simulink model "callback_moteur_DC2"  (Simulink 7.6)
settings: Solver=ode15s  StartTime=0.0  StopTime=N  RelTol=1e-3
InitFcn:
  | % Durée de simulation et temps de l'échelon
  | N=2;
  | t0=N/2;
  | t1=3*N/4;
StopFcn:
  | close all
  | load vit_pos_mot_DC.mat
  | plotyy(x(1,:),x(2,:), x(1,:),x(3,:))
  | grid
  | title('Position et Vitesse d''un moteur DC')
  | gtext('Position (rad)')
  | gtext('Vitesse (rad/s)')
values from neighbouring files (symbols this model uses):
  K = 0.0005    [parametres.m]
  R = 4    [parametres.m]    (also in Prog_callbacks.m = 1000; oscillateur_dephasage.m = 1000; Calcul_Ampl_phase_A.m = 1; circuit_RLC_parallele_.m)
libraries: fl_lib x10, nesl_utility x4

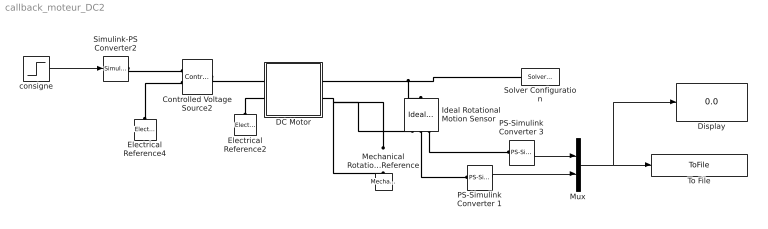
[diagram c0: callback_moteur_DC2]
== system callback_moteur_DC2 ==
  Controlled Voltage Source2 : fl_lib/Electrical/Electrical Sources/Controlled Voltage Source  DialogController=NetworkEngine.DynNeDlgSource  SystemSampleTime=-1  i_Log=off  v_Log=off  LocalVarNames=|current|voltage|power  LocalVarDescs=|Current (A)|Voltage (V)|Power (W)  LocalVarLogging=[0 0 0]
  DC Motor : Subsystem  LoadFcn=|
      | R=4; % Résistance d'induit             
      | L=1e-5; % Inductance d'induit          
      | K=0.0005; % paramètre électromagnétique
  Display : Display
  Electrical Reference2 : fl_lib/Electrical/Electrical Elements/Electrical Reference  DialogController=NetworkEngine.DynNeDlgSource  SystemSampleTime=-1  i_Log=off  LocalVarNames=|i  LocalVarDescs=|i  LocalVarLogging=[]
  Electrical Reference4 : fl_lib/Electrical/Electrical Elements/Electrical Reference  DialogController=NetworkEngine.DynNeDlgSource  SystemSampleTime=-1  i_Log=off  LocalVarNames=|i  LocalVarDescs=|i  LocalVarLogging=[]
  Ideal Rotational Motion Sensor : fl_lib/Mechanical/Mechanical Sensors/Ideal Rotational Motion Sensor  DialogController=NetworkEngine.DynNeDlgSource  SystemSampleTime=-1  offset=0 rad  w_Log=off  t_Log=off  phi_Log=off  LocalVarNames=|w|t|phi  LocalVarDescs=|w|t|phi  LocalVarLogging=[]
  Mechanical Rotational Reference : fl_lib/Mechanical/Rotational Elements/Mechanical Rotational Reference  DialogController=NetworkEngine.DynNeDlgSource  SystemSampleTime=-1  t_Log=off  LocalVarNames=|t  LocalVarDescs=|t  LocalVarLogging=[]
  Mux : Mux  Inputs=2
  PS-Simulink Converter 1 : nesl_utility/PS-Simulink Converter  DialogController=NetworkEngine.DynNeUtilDlgSource  SystemSampleTime=-1  PhysicalDomain=network_engine_domain  LeftPortType=input  RightPortType=output  SubClassName=ps_output  Unit=rpm  AffineConversion=off
  PS-Simulink Converter 3 : nesl_utility/PS-Simulink Converter  DialogController=NetworkEngine.DynNeUtilDlgSource  SystemSampleTime=-1  PhysicalDomain=network_engine_domain  LeftPortType=input  RightPortType=output  SubClassName=ps_output  Unit=rad  AffineConversion=off
  Simulink-PS Converter2 : nesl_utility/Simulink-PS Converter  DialogController=NetworkEngine.DynNeUtilDlgSource  SystemSampleTime=-1  PhysicalDomain=network_engine_domain  LeftPortType=input  RightPortType=output  SubClassName=ps_input  Unit=1  AffineConversion=off  InputFilterTimeConstant=.001  UdotUserProvided=0
  Solver Configuration : nesl_utility/Solver Configuration  DialogController=NetworkEngine.DynNeUtilDlgSource  SystemSampleTime=-1  PhysicalDomain=network_engine_domain  LeftPortType=input  RightPortType=generic  SubClassName=solver  Accelerate=off  Profile=off  ResidualTolerance=1e-9  MaxNonlinIter=3  MaxModeIter=2  DoFixedCost=off  UseLocalSampling=off  DoDC=off  LinearAlgebra=Sparse  LocalSolverSampleTime=.001  LocalSolverChoice=NE_BACKWARD_EULER_ADVANCER  UseLocalSolver=off
  To File : ToFile  Filename=vit_pos_mot_DC.mat  MatrixName=x
  consigne : Step  Time=0.2  After=12  SampleTime=0
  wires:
  PS-Simulink Converter 3/1 -> Mux/1
  PS-Simulink Converter 1/1 -> Mux/2
  Mux/1 -> To File/1, Display/1
  consigne/1 -> Simulink-PS Converter2/1
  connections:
  Electrical Reference2/LConn1 -- DC Motor/LConn2
  DC Motor/RConn2 -- Ideal Rotational Motion Sensor/RConn1 -- Mechanical Rotational Reference/LConn1
  DC Motor/RConn1 -- Solver Configuration/RConn1 -- Ideal Rotational Motion Sensor/LConn1
  Ideal Rotational Motion Sensor/RConn2 -- PS-Simulink Converter 1/LConn1
  Ideal Rotational Motion Sensor/RConn3 -- PS-Simulink Converter 3/LConn1
  Electrical Reference4/LConn1 -- Controlled Voltage Source2/RConn2
  Simulink-PS Converter2/RConn1 -- Controlled Voltage Source2/RConn1
  Controlled Voltage Source2/LConn1 -- DC Motor/LConn1

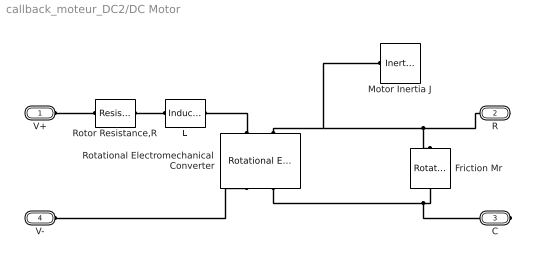
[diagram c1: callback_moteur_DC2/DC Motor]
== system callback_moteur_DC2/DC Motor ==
  Friction Mr : fl_lib/Mechanical/Rotational Elements/Rotational Friction  DialogController=NetworkEngine.DynNeDlgSource  SystemSampleTime=-1  brkwy_trq=0.02e-3 N*m  Col_trq=0.02e-3 N*m  visc_coef=0 N*m/(rad/s)  trans_coef=10 s/rad  vel_thr=0.1 rad/s  t_Log=off  w_Log=off  LocalVarNames=|friction_torque|rel_velocity|power  LocalVarDescs=|Friction torque (N*m)|Relative velocity (rad/s)|Power (W)  LocalVarLogging=[0 0 0]
  L : fl_lib/Electrical/Electrical Elements/Inductor  DialogController=NetworkEngine.DynNeDlgSource  SystemSampleTime=-1  l=L H  i0=0 A  r=0 Ohm  g=1e-09 1/Ohm  i_Log=off  v_Log=off  i_L_Log=off  LocalVarNames=|current|voltage|power  LocalVarDescs=|Inductor current (A) |Voltage across inductor (V)|Power (W)  LocalVarLogging=[0 0 0]
  Motor Inertia J : fl_lib/Mechanical/Rotational Elements/Inertia  DialogController=NetworkEngine.DynNeDlgSource  SystemSampleTime=-1  inertia=0.01 g*cm^2  initial_velocity=0 rad/s  t_Log=off  LocalVarNames=|torque|velocity  LocalVarDescs=|Inertia torque (N*m)|Inertia absolute velocity (rad/s)  LocalVarLogging=[0 0]
  Rotational Electromechanical Converter : fl_lib/Electrical/Electrical Elements/Rotational Electromechanical Converter  DialogController=NetworkEngine.DynNeDlgSource  SystemSampleTime=-1  K=K V/(rad/s)  i_Log=off  v_Log=off  t_Log=off  w_Log=off  LocalVarNames=|current|voltage|power|torque|speed  LocalVarDescs=|Current (A)|Voltage (V)|Power (W)|Torque (Nm)|Angular speed (rad/s)  LocalVarLogging=[0 0 0 0 0]
  Rotor Resistance,R : fl_lib/Electrical/Electrical Elements/Resistor  Tag=Factory Generic  DialogController=NetworkEngine.DynNeDlgSource  SystemSampleTime=-1  R=R Ohm  i_Log=off  v_Log=off  LocalVarNames=|current|voltage|power  LocalVarDescs=|Resistor current (A)|Voltage across resistor (V)|Power (W)  LocalVarLogging=[0 0 0]
  V+ : PMIOPort  Port=1  Side=Left
  R : PMIOPort  Port=2  Side=Right
  C : PMIOPort  Port=3  Side=Right
  V- : PMIOPort  Port=4  Side=Left
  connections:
  Rotational Electromechanical Converter/LConn1 -- L/RConn1
  V-/RConn1 -- Rotational Electromechanical Converter/RConn1
  Rotor Resistance,R/LConn1 -- V+/RConn1
  L/LConn1 -- Rotor Resistance,R/RConn1
  Rotational Electromechanical Converter/LConn2 -- R/RConn1 -- Friction Mr/LConn1 -- Motor Inertia J/LConn1
  Rotational Electromechanical Converter/RConn2 -- C/RConn1 -- Friction Mr/RConn1
